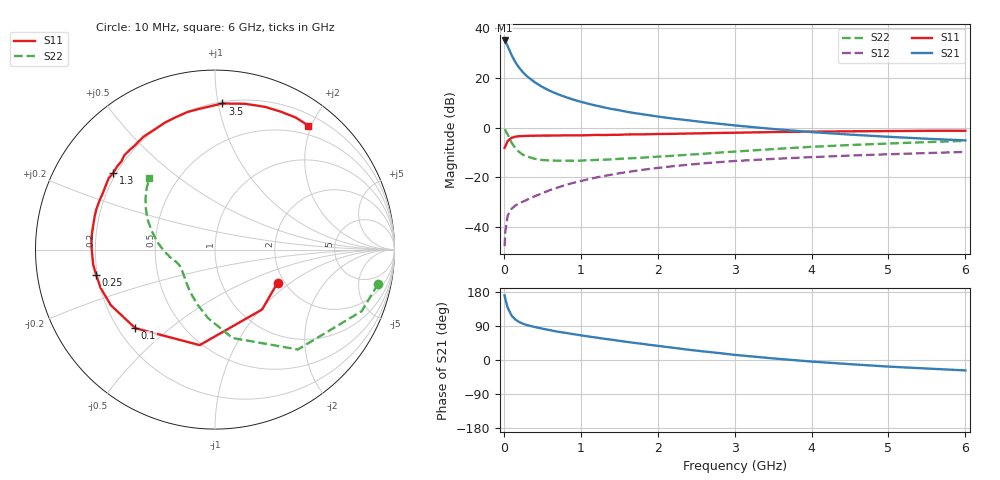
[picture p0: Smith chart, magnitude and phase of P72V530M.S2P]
! SIEMENS Small Signal Semiconductors
! BFP196
! Si NPN RF Bipolar Junction Transistor in SOT143
! VCE = 2.5 V  IC = 30 mA
! Common Emitter S-Parameters:  May  1996
# GHz  S  MA  R  50
!  f  S11  S21  S12  S22
! GHz  MAG  ANG  MAG  ANG  MAG  ANG  MAG  ANG
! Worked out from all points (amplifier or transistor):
!   36 points, 10 MHz to 6 GHz, reference 50 ohm
!   highest |S21| = 34.9 dB at 10 MHz (marker M1)
!   |S21| within 3 dB of that: start of sweep to 60.17 MHz
!   unconditionally stable (mu >= 1): 544.6 MHz to 3.788 GHz
!   at 250 MHz: K = 0.73, MSG = 25.9 dB, |S12| = -29.7 dB
!   at 1.4 GHz: K = 1.10, MAG = 11.2 dB, |S12| = -18.9 dB
!   at 6 GHz: K = 0.97, MSG = 2.3 dB, |S12| = -9.8 dB
!   lowest NFmin = 1.40 dB at 500 MHz
!   S11 on the Smith chart (normalised r, x): 10 MHz: 1.84, -0.80; 100 MHz: 0.27, -0.38; 250 MHz: 0.19, -0.10; 1.3 GHz: 0.19, +0.32; 3.5 GHz: 0.21, +1.03; 6 GHz: 0.36, +1.95
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0.01  0.3942 -27.8  55.81 170.4  0.0042 79.9  0.9285 -11.9
0.02  0.4246 -51.8  53.24 160.0  0.0084 73.9  0.8867 -22.7
0.05  0.539 -99.1  42.93 138.0  0.0173 57.0  0.7233 -50.3
0.1  0.6237 -135.4  28.53 117.4  0.0235 47.0  0.502 -78.8
0.15  0.6578 -151.9  20.43 106.7  0.0275 43.9  0.3847 -95.6
0.2  0.672 -161.4  15.82 100.1  0.0302 45.2  0.3228 -107.4
0.25  0.6769 -168.1  12.75 95.6  0.0329 46.7  0.2846 -116.7
0.3  0.6839 -172.8  10.74 92.3  0.0357 49.3  0.2634 -123.5
0.4  0.6873 179.6  8.144 87.1  0.042 52.4  0.237 -134.1
0.5  0.692 174.6  6.524 82.8  0.0483 55.1  0.2243 -141.2
0.6  0.6917 169.4  5.45 78.7  0.056 56.1  0.219 -146.1
0.7  0.6952 164.9  4.683 74.7  0.063 57.4  0.2174 -149.9
0.9  0.6991 157.1  3.651 68.3  0.0778 57.5  0.2164 -155.7
1.1  0.705 149.9  3.003 62.1  0.0923 57.0  0.2216 -159.4
1.3  0.7098 143.1  2.548 56.2  0.1072 55.1  0.2273 -162.8
1.7  0.7309 130.4  1.953 45.1  0.135 51.1  0.2446 -168.7
2.2  0.7492 116.7  1.517 32.3  0.1683 44.7  0.2724 -175.6
3  0.7884 96.8  1.106 13.6  0.2137 33.8  0.3301 171.1
3.5  0.8151 87.1  0.938 4.2  0.2357 27.1  0.3707 163.0
4.5  0.8427 70.7  0.724 -11.0  0.2749 15.6  0.447 149.5
5.5  0.8625 58.5  0.598 -22.5  0.309 4.7  0.512 138.0
6  0.8647 53.0  0.554 -27.5  0.3252 -1.1  0.5413 132.4
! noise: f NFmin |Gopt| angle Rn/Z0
0.5  1.4  0.4  -173  0.08
0.9  1.6  0.5  -166  0.08
1.5  2.4  0.61  -150  0.14
2  2.9  0.71  -129  0.2
